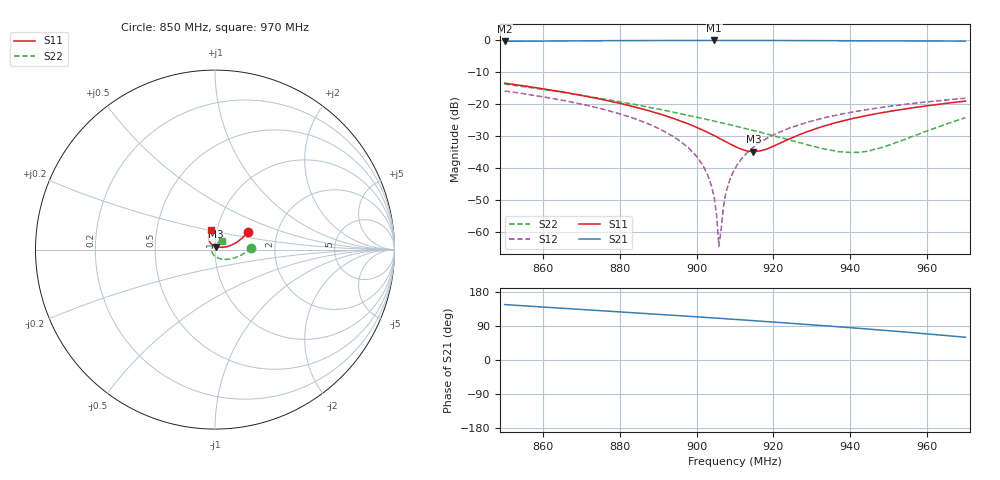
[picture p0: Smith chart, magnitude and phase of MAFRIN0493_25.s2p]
!Part Number:  MAFRIN0493
!Name:  MC
!Comments:  1
!Thu 09/Dec/2004  2:37:29 PM
!Temperature:  25
# MHZ  S  DB  R  50
!Freq  S11(dB)  S11(ang)  S21(dB)  S21(ang)  S12(dB)  S12(ang)  S22(dB)  S22(ang)
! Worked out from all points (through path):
!   201 points, 850 MHz to 970 MHz, reference 50 ohm
!   highest |S21| = -0.22 dB at 904.6 MHz (marker M1); lowest = -0.5 dB at 850 MHz (marker M2)
!   group delay of S21, straight-line fit = 1.97 ns
!   lowest |S11| = -35.0 dB at 914.8 MHz (marker M3), VSWR 1.04, Z = 50.5 + j1.71 ohm
!   |S11| at or under -10 dB: start of sweep to end of sweep
!   |S22| runs from -35.3 to -13.9 dB; largest |S21 - S12| = 1.1
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850  -13.59 28.6  -0.49 146.2  -16.04 102.7  -13.87 3.0
870.4  -17.49 19.1  -0.32 133.4  -20.24 87.8  -17.44 -16.8
881.8  -20.42 15.3  -0.27 126.1  -23.85 79.9  -19.81 -30.1
890.2  -23.14 13.9  -0.24 120.6  -27.81 74.4  -21.74 -41.4
895.6  -25.34 14.7  -0.24 117.0  -31.62 71.1  -23.09 -49.9
899.8  -27.31 17.3  -0.23 114.1  -36.22 68.8  -24.16 -56.8
902.8  -28.94 20.8  -0.23 112.1  -42.08 68.8  -24.95 -62.3
904.6  -30.00 23.9  -0.22 110.9  -49.42 71.6  -25.43 -65.6
905.2  -30.33 25.1  -0.23 110.5  -54.83 75.1  -25.61 -66.8
905.8  -30.75 26.6  -0.23 110.0  -64.57 105.8  -25.80 -67.9
906.4  -31.12 28.3  -0.23 109.6  -59.15 -138.1  -25.97 -69.1
907  -31.50 29.7  -0.23 109.2  -52.08 -125.4  -26.12 -70.4
907.6  -31.90 31.8  -0.23 108.8  -47.92 -123.0  -26.28 -71.7
908.8  -32.65 36.4  -0.23 108.0  -43.36 -121.0  -26.61 -74.3
910  -33.38 41.7  -0.23 107.1  -40.38 -121.2  -26.98 -76.7
911.8  -34.27 52.2  -0.23 105.9  -37.14 -121.8  -27.54 -80.8
914.8  -35.01 72.7  -0.23 103.8  -33.63 -122.8  -28.42 -88.1
922  -32.20 110.4  -0.24 98.7  -28.67 -126.7  -30.65 -107.9
930.4  -28.08 123.6  -0.26 92.5  -25.29 -131.6  -33.31 -138.3
940.6  -24.66 123.7  -0.29 84.8  -22.60 -137.6  -35.30 167.6
950.2  -22.42 118.8  -0.33 77.2  -20.82 -143.2  -32.95 112.7
970  -19.19 100.8  -0.42 60.0  -18.29 -153.7  -24.38 50.8
